(* Logix 5000 AddOnInstructionDefinition export SPEL_LocalGet; software revision 30.01 *)

ADD_ON_INSTRUCTION SPEL_ExecCmd   (* revision 1.2 *)
// Executes a command in the robot controller.  Normally this is called by higher level AOIs.
VAR_INPUT
   Start : BOOL; {required}
   MaxTime : DINT := 3000; {required}
END_VAR
VAR_OUTPUT
   InCycle : BOOL; {access Read Only, visible}
   Done : BOOL; {access Read Only, visible}
   Error : BOOL; {access Read Only, visible}
END_VAR
VAR_IN_OUT
   ExtInputs : AB:ETHERNET_MODULE_INT_128Bytes:I:0; {required}
        .DATA[0].0   // ExtCmdGet
        .DATA[0].1   // ExtRespSet
        .DATA[0].2   // ExtCmdResult
        .DATA[0].3   // ExtError
   ExtOutputs : AB:ETHERNET_MODULE_INT_128Bytes:O:0; {required}
        .DATA[0].0   // ExtCmdSet
        .DATA[0].1   // ExtRespGet
        .DATA[0].2   // ExtCmdReset
END_VAR
VAR_INPUT
   Cmd : INT; {required}
   CmdParam1 : INT; {required}
   CmdParam2 : INT; {required}
   CmdParam3 : INT; {required}
   CmdParam4 : INT; {required}
   CmdParam5 : INT; {required}
   CmdParam6 : INT; {required}
   CmdParam7 : INT; {required}
END_VAR
VAR_OUTPUT
   CmdEcho : INT; {access Read Only, visible}
   Resp1 : INT; {access Read Only, visible}
   Resp2 : INT; {access Read Only, visible}
   Resp3 : INT; {access Read Only, visible}
   Resp4 : INT; {access Read Only, visible}
   Resp5 : INT; {access Read Only, visible}
   Resp6 : INT; {access Read Only, visible}
   Resp7 : INT; {access Read Only, visible}
   ErrCode1 : INT; {access Read Only, visible}
   ErrCode2 : INT; {access Read Only, visible}
END_VAR
VAR
   ExtReset : BOOL; {access None}
   ExtError : BOOL; {access None}
   ExtCmdSet : BOOL; {access None}   // Cmd Ready
   ExtCmdGet : BOOL; {access None}   // Cmd Received
   CmdXferDone : BOOL; {access None}
   ExtRespSet : BOOL; {access None}   // Resp Ready
   RespXferDone : BOOL; {access None}
   ExtCmdResult : BOOL; {access None}   // Normal or Error?
   TmrCmdDataRdy : TIMER := (PRE := 5); {access None}
   OneShotDoneOff : BOOL; {access None}
   OneShotStart : BOOL; {access None}
   StartInit : BOOL; {access None}
   OneShotStartError : BOOL; {access None}
   TmrCycle : TIMER := (PRE := 5000); {access None}
   OneshotTmrPreset : BOOL; {access None}
   TmrCmdSet : TIMER := (PRE := 20); {access None}
   OnShotCmdDataXfer : BOOL; {access None}
   OneShotRespDataXfer : BOOL; {access None}
   OneShotDataRdy : BOOL; {access None}
   OtherCmdInCycle : BOOL; {access None}
   s : BOOL; {access None}
   OneShotUnsetCmdIncycle : BOOL; {access None}
   OneShotSetCmdIncycle : BOOL; {access None}
   OneShotSetOtherCmdInCycleError : BOOL; {access None}
   OneShotSetBit : BOOL; {access None}
   MaxTimeError : BOOL; {access None}
END_VAR

ROUTINE Logic   (* ladder *)
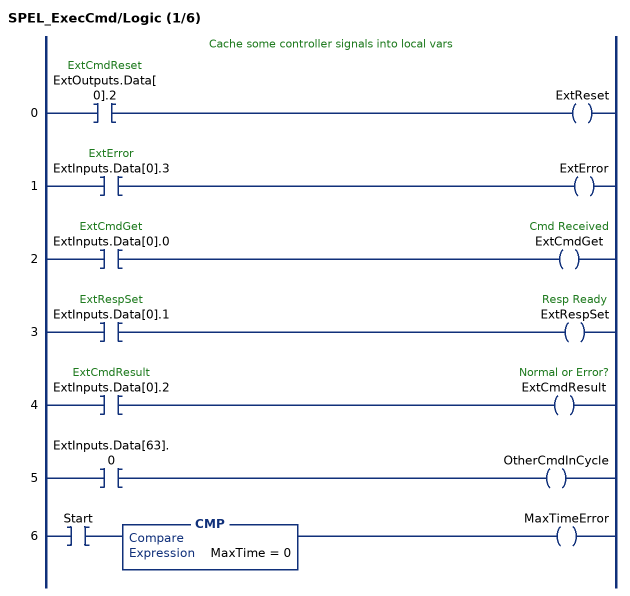
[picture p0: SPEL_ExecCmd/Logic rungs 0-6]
   // Cache some controller signals into local vars
   0: XIC(ExtOutputs.Data[0].2)OTE(ExtReset);
   1: XIC(ExtInputs.Data[0].3)OTE(ExtError);
   2: XIC(ExtInputs.Data[0].0)OTE(ExtCmdGet);
   3: XIC(ExtInputs.Data[0].1)OTE(ExtRespSet);
   4: XIC(ExtInputs.Data[0].2)OTE(ExtCmdResult);
   5: XIC(ExtInputs.Data[63].0)OTE(OtherCmdInCycle);
   6: XIC(Start)CMP(MaxTime = 0)OTE(MaxTimeError);
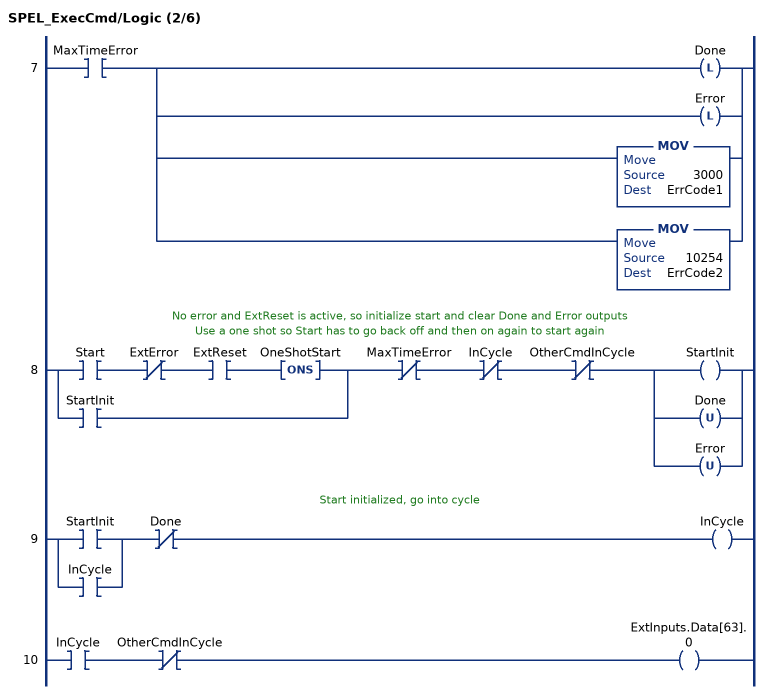
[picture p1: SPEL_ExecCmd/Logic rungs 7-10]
   7: XIC(MaxTimeError)[OTL(Done) ,OTL(Error) ,MOV(3000,ErrCode1) ,MOV(10254,ErrCode2) ];
   // No error and ExtReset is active, so initialize start and clear Done and Error outputs
   // Use a one shot so Start has to go back off and then on again to start again
   8: [XIC(Start) XIO(ExtError) XIC(ExtReset) ONS(OneShotStart) ,XIC(StartInit) ]XIO(MaxTimeError)XIO(InCycle)XIO(OtherCmdInCycle)[OTE(StartInit) ,OTU(Done) ,OTU(Error) ];
   // Start initialized, go into cycle
   9: [XIC(StartInit) ,XIC(InCycle) ]XIO(Done)OTE(InCycle);
   10: XIC(InCycle)XIO(OtherCmdInCycle)OTE(ExtInputs.Data[63].0);
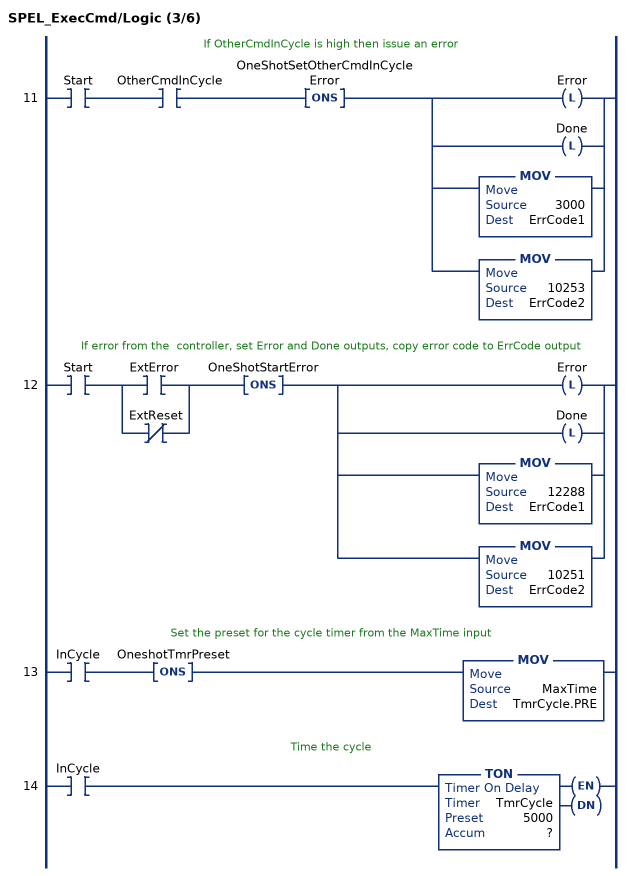
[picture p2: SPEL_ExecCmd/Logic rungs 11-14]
   // If OtherCmdInCycle is high then issue an error
   11: XIC(Start)XIC(OtherCmdInCycle)ONS(OneShotSetOtherCmdInCycleError)[OTL(Error) ,OTL(Done) ,MOV(3000,ErrCode1) ,MOV(10253,ErrCode2) ];
   // If error from the  controller, set Error and Done outputs, copy error code to ErrCode output
   12: XIC(Start)[XIC(ExtError) ,XIO(ExtReset) ]ONS(OneShotStartError)[OTL(Error) ,OTL(Done) ,MOV(12288,ErrCode1) ,MOV(10251,ErrCode2) ];
   // Set the preset for the cycle timer from the MaxTime input
   13: XIC(InCycle)ONS(OneshotTmrPreset)MOV(MaxTime,TmrCycle.PRE);
   // Time the cycle
   14: XIC(InCycle)TON(TmrCycle,?,?);
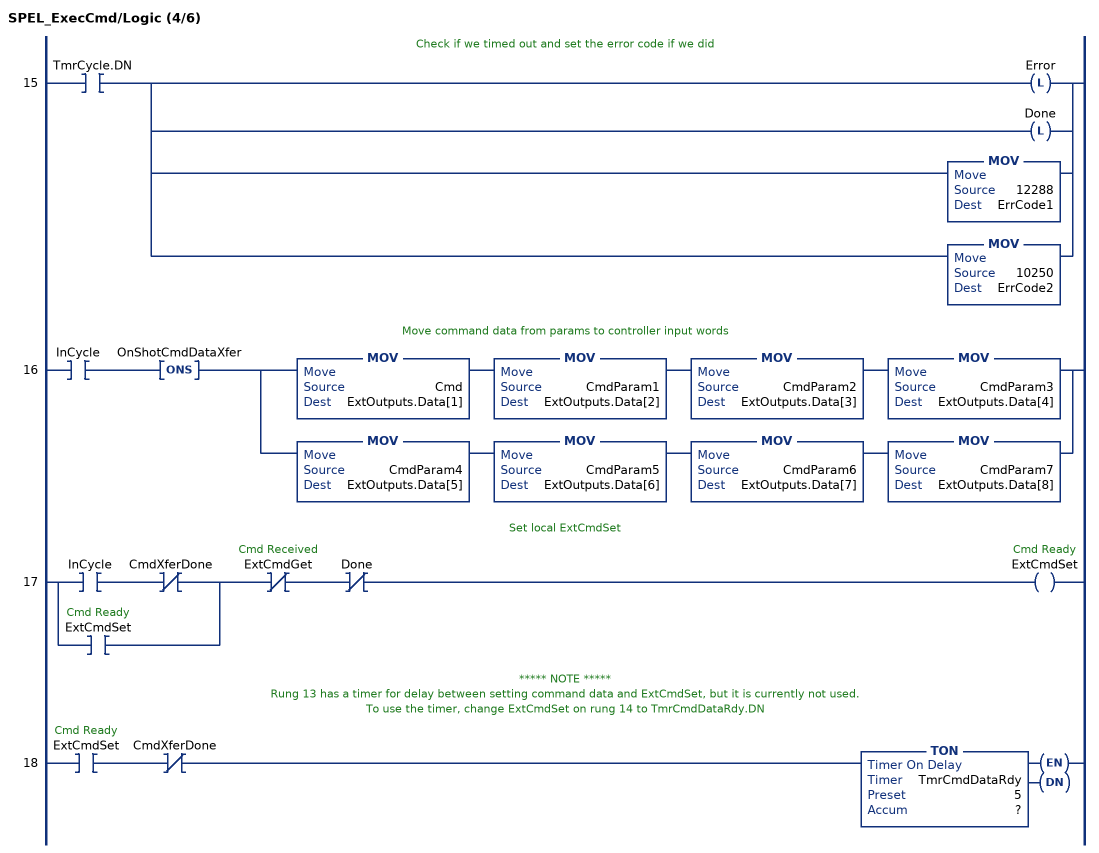
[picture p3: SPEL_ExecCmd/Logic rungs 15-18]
   // Check if we timed out and set the error code if we did
   15: XIC(TmrCycle.DN)[OTL(Error) ,OTL(Done) ,MOV(12288,ErrCode1) ,MOV(10250,ErrCode2) ];
   // Move command data from params to controller input words
   16: XIC(InCycle)ONS(OnShotCmdDataXfer)[MOV(Cmd,ExtOutputs.Data[1]) MOV(CmdParam1,ExtOutputs.Data[2]) MOV(CmdParam2,ExtOutputs.Data[3]) MOV(CmdParam3,ExtOutputs.Data[4]) ,MOV(CmdParam4,ExtOutputs.Data[5]) MOV(CmdParam5,ExtOutputs.Data[6]) MOV(CmdParam6,ExtOutputs.Data[7]) MOV(CmdParam7,ExtOutputs.Data[8]) ];
   // Set local ExtCmdSet
   17: [XIC(InCycle) XIO(CmdXferDone) ,XIC(ExtCmdSet) ]XIO(ExtCmdGet)XIO(Done)OTE(ExtCmdSet);
   // ***** NOTE *****
   // Rung 13 has a timer for delay between setting command data and ExtCmdSet, but it is currently not used.
   // To use the timer, change ExtCmdSet on rung 14 to TmrCmdDataRdy.DN
   18: XIC(ExtCmdSet)XIO(CmdXferDone)TON(TmrCmdDataRdy,?,?);
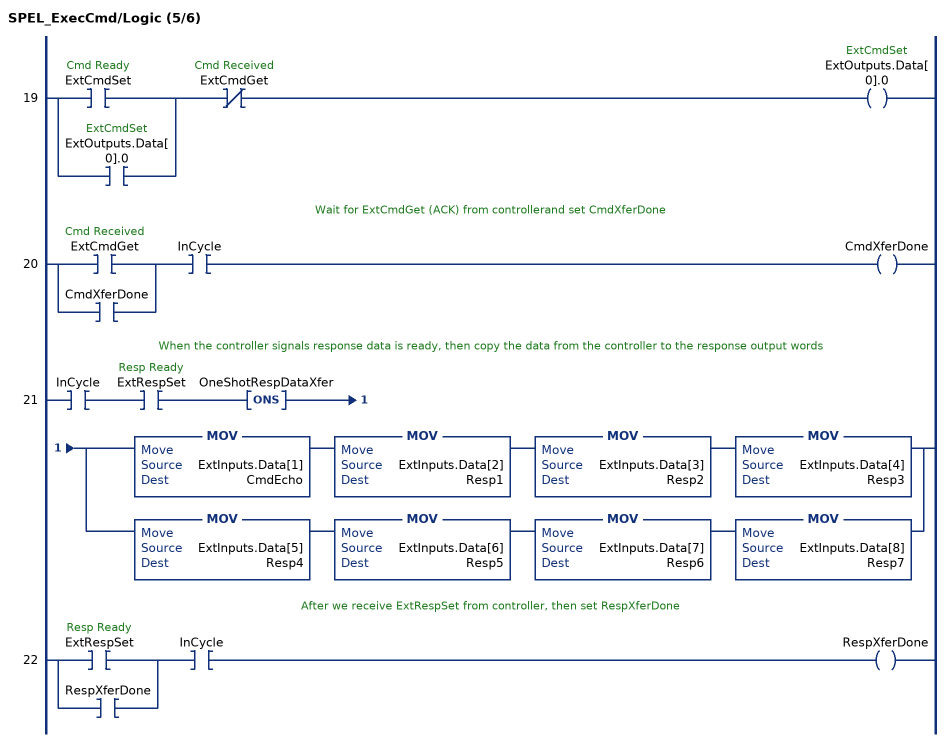
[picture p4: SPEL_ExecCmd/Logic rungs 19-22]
   19: [XIC(ExtCmdSet) ,XIC(ExtOutputs.Data[0].0) ]XIO(ExtCmdGet)OTE(ExtOutputs.Data[0].0);
   // Wait for ExtCmdGet (ACK) from controllerand set CmdXferDone
   20: [XIC(ExtCmdGet) ,XIC(CmdXferDone) ]XIC(InCycle)OTE(CmdXferDone);
   // When the controller signals response data is ready, then copy the data from the controller to the response output words
   21: XIC(InCycle)XIC(ExtRespSet)ONS(OneShotRespDataXfer)[MOV(ExtInputs.Data[1],CmdEcho) MOV(ExtInputs.Data[2],Resp1) MOV(ExtInputs.Data[3],Resp2) MOV(ExtInputs.Data[4],Resp3) ,MOV(ExtInputs.Data[5],Resp4) MOV(ExtInputs.Data[6],Resp5) MOV(ExtInputs.Data[7],Resp6) MOV(ExtInputs.Data[8],Resp7) ];
   // After we receive ExtRespSet from controller, then set RespXferDone
   22: [XIC(ExtRespSet) ,XIC(RespXferDone) ]XIC(InCycle)OTE(RespXferDone);
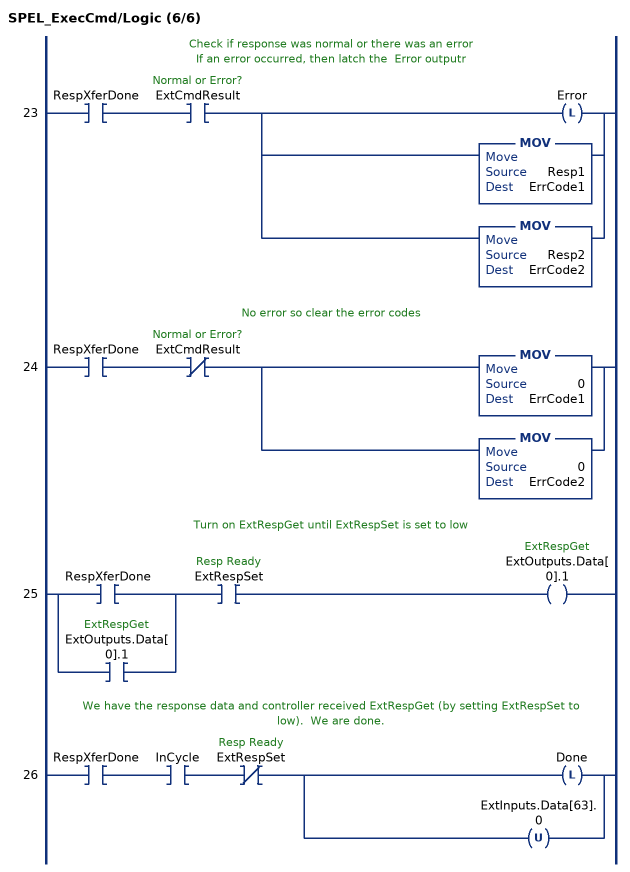
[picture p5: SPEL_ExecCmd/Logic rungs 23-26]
   // Check if response was normal or there was an error
   // If an error occurred, then latch the  Error outputr
   23: XIC(RespXferDone)XIC(ExtCmdResult)[OTL(Error) ,MOV(Resp1,ErrCode1) ,MOV(Resp2,ErrCode2) ];
   // No error so clear the error codes
   24: XIC(RespXferDone)XIO(ExtCmdResult)[MOV(0,ErrCode1) ,MOV(0,ErrCode2) ];
   // Turn on ExtRespGet until ExtRespSet is set to low
   25: [XIC(RespXferDone) ,XIC(ExtOutputs.Data[0].1) ]XIC(ExtRespSet)OTE(ExtOutputs.Data[0].1);
   // We have the response data and controller received ExtRespGet (by setting ExtRespSet to low).  We are done.
   26: XIC(RespXferDone)XIC(InCycle)XIO(ExtRespSet)[OTL(Done) ,OTU(ExtInputs.Data[63].0) ];
END_ROUTINE
END_ADD_ON_INSTRUCTION

ADD_ON_INSTRUCTION SPEL_LocalGet   (* revision 1.2, vendor SEIKO EPSON CORP. *)
// Gets the setting status of the Local coordinate system number.
VAR_INPUT
   Start : BOOL; {required}
END_VAR
VAR_OUTPUT
   InCycle : BOOL; {access Read Only, visible}
   Done : BOOL; {access Read Only, visible}
   Error : BOOL; {access Read Only, visible}
END_VAR
VAR_INPUT
   NumAxes : INT; {required}
   LocalNum : INT; {required}
END_VAR
VAR_OUTPUT
   LocalX : REAL; {visible}
   LocalY : REAL; {visible}
   LocalZ : REAL; {visible}
   LocalU : REAL; {visible}
   LocalV : REAL; {visible}
   LocalW : REAL; {visible}
END_VAR
VAR_IN_OUT
   ExtInputs : AB:ETHERNET_MODULE_INT_128Bytes:I:0; {required}
   ExtOutputs : AB:ETHERNET_MODULE_INT_128Bytes:O:0; {required}
END_VAR
VAR_OUTPUT
   ErrCode1 : INT; {access Read Only, visible}
   ErrCode2 : INT; {access Read Only, visible}
END_VAR
VAR
   Coordinatex1000 : DINT; {access None}
   Coordinate_INTS : INT[2]; {access None}
   ExecLocalGetZ : SPEL_ExecCmd := (MaxTime := 3000); {access None}
   ExecLocalGetY : SPEL_ExecCmd := (MaxTime := 3000); {access None}
   ExecLocalGetX : SPEL_ExecCmd := (MaxTime := 3000); {access None}
   X6 : BOOL; {access None}
   StartInit : BOOL[32]; {access None}
   OneShotStart : BOOL[32]; {access None}
   ExecLocalGetW : SPEL_ExecCmd := (MaxTime := 3000); {access None}
   ExecLocalGetV : SPEL_ExecCmd := (MaxTime := 3000); {access None}
   ExecLocalGetU : SPEL_ExecCmd := (MaxTime := 3000); {access None}
   ExecTimeout : DINT; {access None}
END_VAR

ROUTINE Logic   (* ladder *)
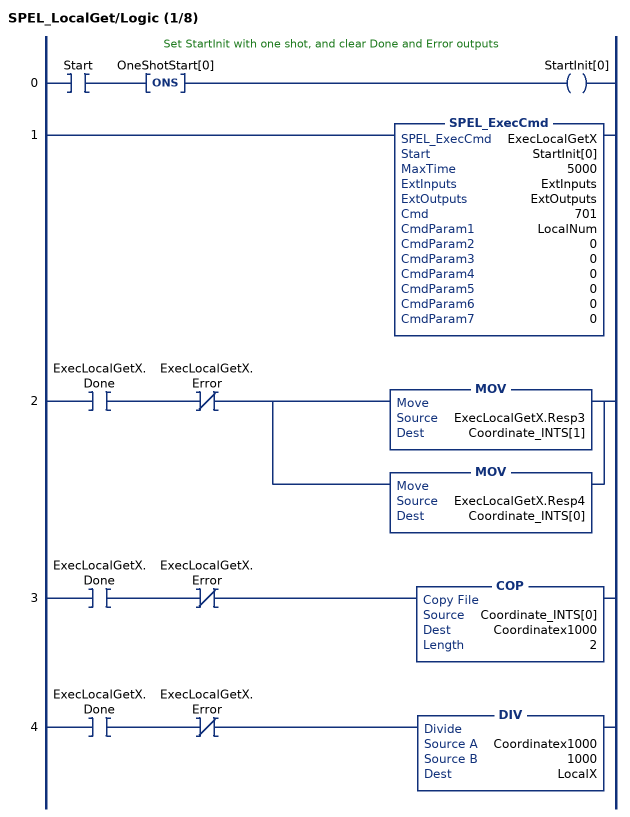
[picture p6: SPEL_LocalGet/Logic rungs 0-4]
   // Set StartInit with one shot, and clear Done and Error outputs
   0: XIC(Start)ONS(OneShotStart[0])OTE(StartInit[0]);
   1: SPEL_ExecCmd(ExecLocalGetX,StartInit[0],5000,ExtInputs,ExtOutputs,701,LocalNum,0,0,0,0,0,0);
   2: XIC(ExecLocalGetX.Done)XIO(ExecLocalGetX.Error)[MOV(ExecLocalGetX.Resp3,Coordinate_INTS[1]) ,MOV(ExecLocalGetX.Resp4,Coordinate_INTS[0]) ];
   3: XIC(ExecLocalGetX.Done)XIO(ExecLocalGetX.Error)COP(Coordinate_INTS[0],Coordinatex1000,2);
   4: XIC(ExecLocalGetX.Done)XIO(ExecLocalGetX.Error)DIV(Coordinatex1000,1000,LocalX);
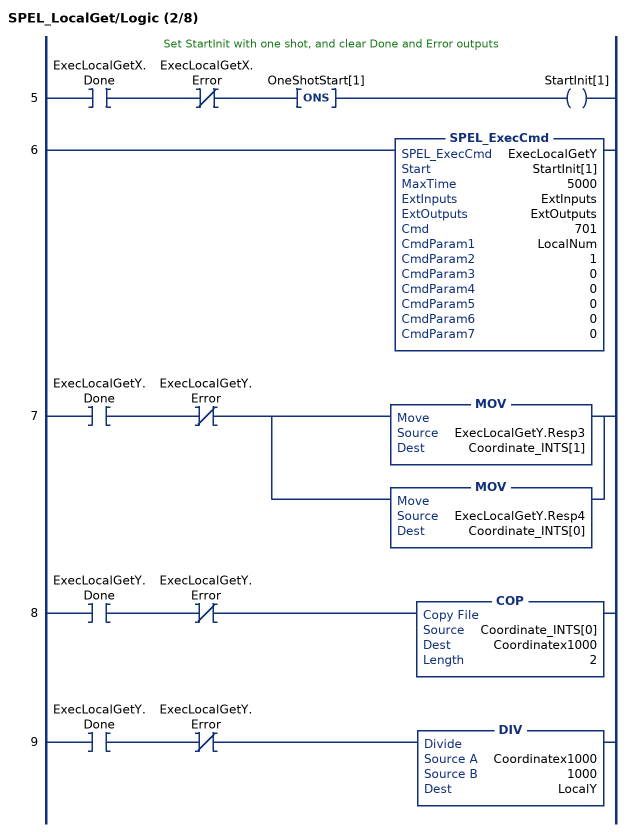
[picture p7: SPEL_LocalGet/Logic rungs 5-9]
   // Set StartInit with one shot, and clear Done and Error outputs
   5: XIC(ExecLocalGetX.Done)XIO(ExecLocalGetX.Error)ONS(OneShotStart[1])OTE(StartInit[1]);
   6: SPEL_ExecCmd(ExecLocalGetY,StartInit[1],5000,ExtInputs,ExtOutputs,701,LocalNum,1,0,0,0,0,0);
   7: XIC(ExecLocalGetY.Done)XIO(ExecLocalGetY.Error)[MOV(ExecLocalGetY.Resp3,Coordinate_INTS[1]) ,MOV(ExecLocalGetY.Resp4,Coordinate_INTS[0]) ];
   8: XIC(ExecLocalGetY.Done)XIO(ExecLocalGetY.Error)COP(Coordinate_INTS[0],Coordinatex1000,2);
   9: XIC(ExecLocalGetY.Done)XIO(ExecLocalGetY.Error)DIV(Coordinatex1000,1000,LocalY);
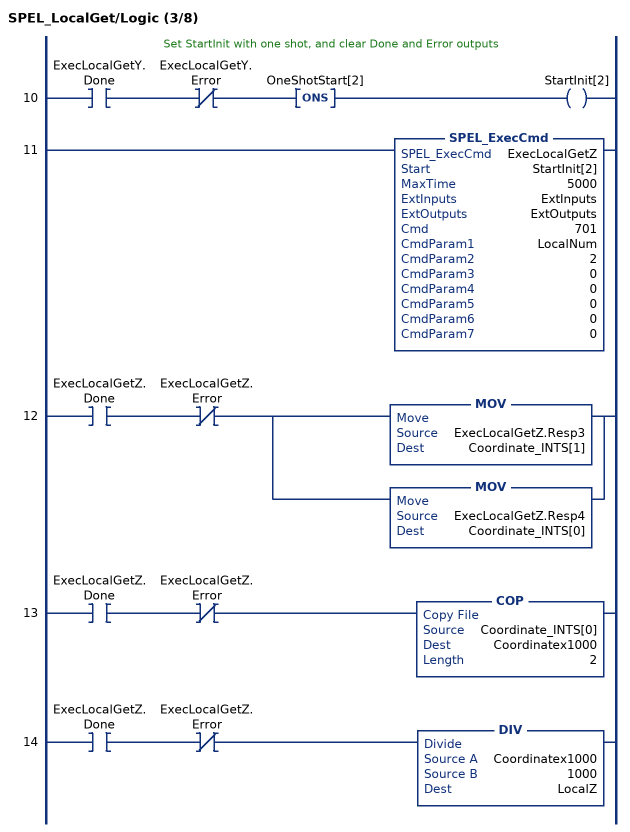
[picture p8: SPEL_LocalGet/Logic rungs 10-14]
   // Set StartInit with one shot, and clear Done and Error outputs
   10: XIC(ExecLocalGetY.Done)XIO(ExecLocalGetY.Error)ONS(OneShotStart[2])OTE(StartInit[2]);
   11: SPEL_ExecCmd(ExecLocalGetZ,StartInit[2],5000,ExtInputs,ExtOutputs,701,LocalNum,2,0,0,0,0,0);
   12: XIC(ExecLocalGetZ.Done)XIO(ExecLocalGetZ.Error)[MOV(ExecLocalGetZ.Resp3,Coordinate_INTS[1]) ,MOV(ExecLocalGetZ.Resp4,Coordinate_INTS[0]) ];
   13: XIC(ExecLocalGetZ.Done)XIO(ExecLocalGetZ.Error)COP(Coordinate_INTS[0],Coordinatex1000,2);
   14: XIC(ExecLocalGetZ.Done)XIO(ExecLocalGetZ.Error)DIV(Coordinatex1000,1000,LocalZ);
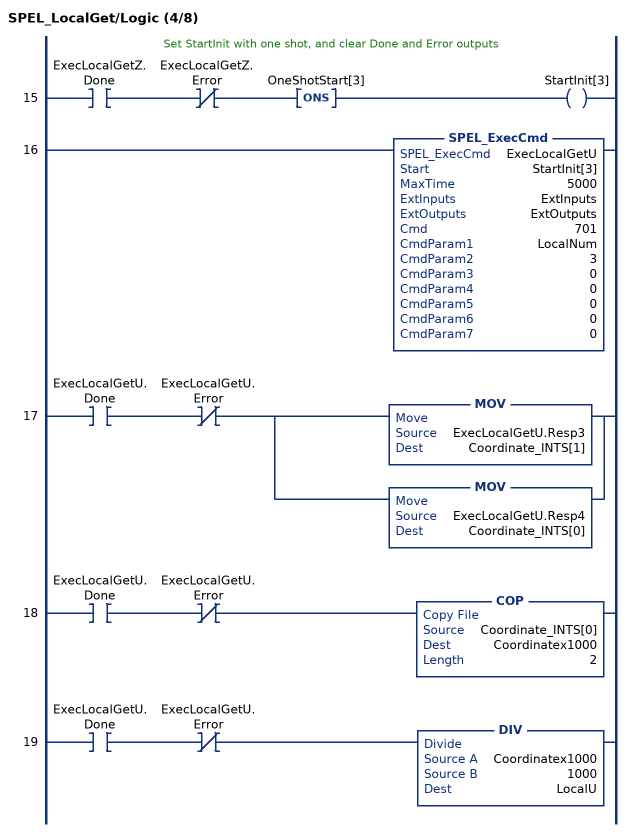
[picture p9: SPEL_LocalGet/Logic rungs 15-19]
   // Set StartInit with one shot, and clear Done and Error outputs
   15: XIC(ExecLocalGetZ.Done)XIO(ExecLocalGetZ.Error)ONS(OneShotStart[3])OTE(StartInit[3]);
   16: SPEL_ExecCmd(ExecLocalGetU,StartInit[3],5000,ExtInputs,ExtOutputs,701,LocalNum,3,0,0,0,0,0);
   17: XIC(ExecLocalGetU.Done)XIO(ExecLocalGetU.Error)[MOV(ExecLocalGetU.Resp3,Coordinate_INTS[1]) ,MOV(ExecLocalGetU.Resp4,Coordinate_INTS[0]) ];
   18: XIC(ExecLocalGetU.Done)XIO(ExecLocalGetU.Error)COP(Coordinate_INTS[0],Coordinatex1000,2);
   19: XIC(ExecLocalGetU.Done)XIO(ExecLocalGetU.Error)DIV(Coordinatex1000,1000,LocalU);
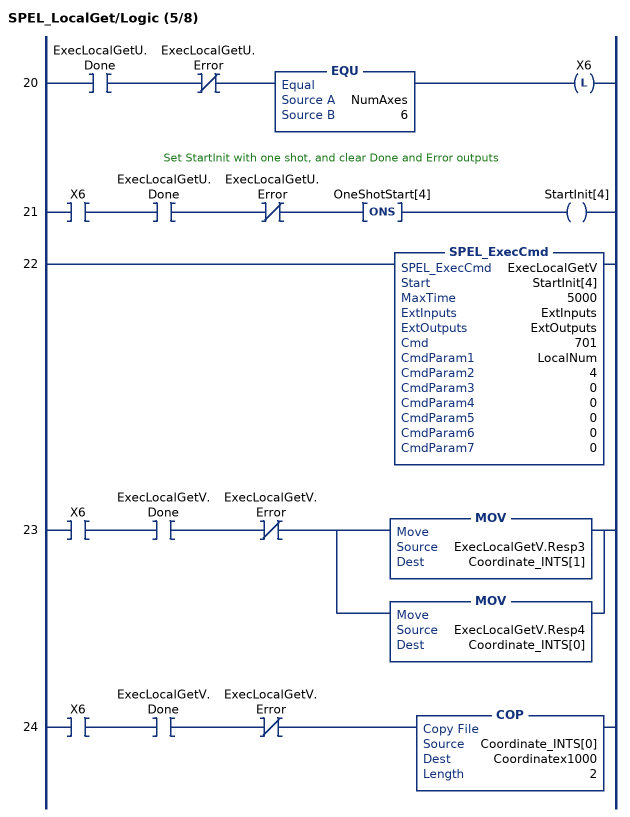
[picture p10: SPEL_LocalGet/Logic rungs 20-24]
   20: XIC(ExecLocalGetU.Done)XIO(ExecLocalGetU.Error)EQU(NumAxes,6)OTL(X6);
   // Set StartInit with one shot, and clear Done and Error outputs
   21: XIC(X6)XIC(ExecLocalGetU.Done)XIO(ExecLocalGetU.Error)ONS(OneShotStart[4])OTE(StartInit[4]);
   22: SPEL_ExecCmd(ExecLocalGetV,StartInit[4],5000,ExtInputs,ExtOutputs,701,LocalNum,4,0,0,0,0,0);
   23: XIC(X6)XIC(ExecLocalGetV.Done)XIO(ExecLocalGetV.Error)[MOV(ExecLocalGetV.Resp3,Coordinate_INTS[1]) ,MOV(ExecLocalGetV.Resp4,Coordinate_INTS[0]) ];
   24: XIC(X6)XIC(ExecLocalGetV.Done)XIO(ExecLocalGetV.Error)COP(Coordinate_INTS[0],Coordinatex1000,2);
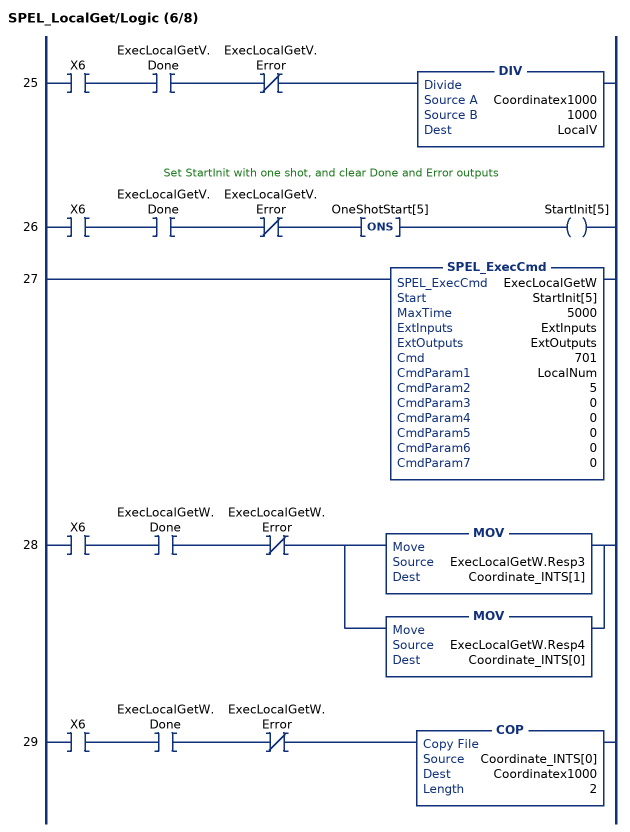
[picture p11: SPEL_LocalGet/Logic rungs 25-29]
   25: XIC(X6)XIC(ExecLocalGetV.Done)XIO(ExecLocalGetV.Error)DIV(Coordinatex1000,1000,LocalV);
   // Set StartInit with one shot, and clear Done and Error outputs
   26: XIC(X6)XIC(ExecLocalGetV.Done)XIO(ExecLocalGetV.Error)ONS(OneShotStart[5])OTE(StartInit[5]);
   27: SPEL_ExecCmd(ExecLocalGetW,StartInit[5],5000,ExtInputs,ExtOutputs,701,LocalNum,5,0,0,0,0,0);
   28: XIC(X6)XIC(ExecLocalGetW.Done)XIO(ExecLocalGetW.Error)[MOV(ExecLocalGetW.Resp3,Coordinate_INTS[1]) ,MOV(ExecLocalGetW.Resp4,Coordinate_INTS[0]) ];
   29: XIC(X6)XIC(ExecLocalGetW.Done)XIO(ExecLocalGetW.Error)COP(Coordinate_INTS[0],Coordinatex1000,2);
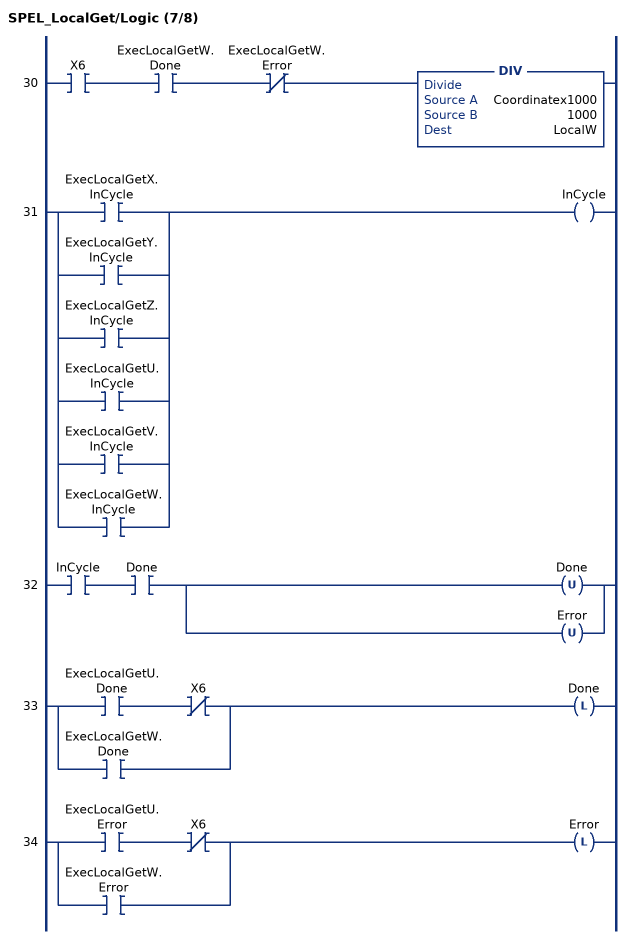
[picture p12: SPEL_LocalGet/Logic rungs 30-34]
   30: XIC(X6)XIC(ExecLocalGetW.Done)XIO(ExecLocalGetW.Error)DIV(Coordinatex1000,1000,LocalW);
   31: [XIC(ExecLocalGetX.InCycle) ,XIC(ExecLocalGetY.InCycle) ,XIC(ExecLocalGetZ.InCycle) ,XIC(ExecLocalGetU.InCycle) ,XIC(ExecLocalGetV.InCycle) ,XIC(ExecLocalGetW.InCycle) ]OTE(InCycle);
   32: XIC(InCycle)XIC(Done)[OTU(Done) ,OTU(Error) ];
   33: [XIC(ExecLocalGetU.Done) XIO(X6) ,XIC(ExecLocalGetW.Done) ]OTL(Done);
   34: [XIC(ExecLocalGetU.Error) XIO(X6) ,XIC(ExecLocalGetW.Error) ]OTL(Error);
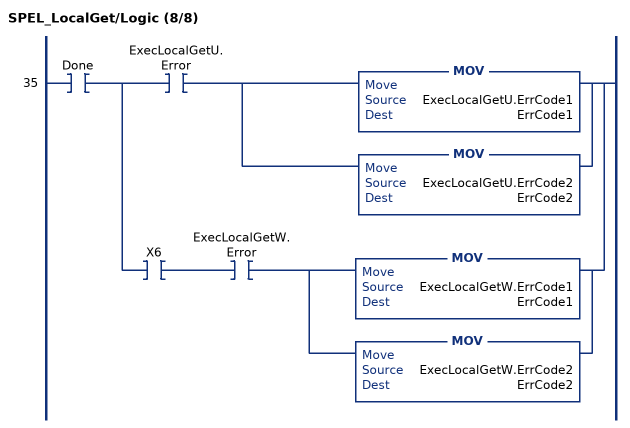
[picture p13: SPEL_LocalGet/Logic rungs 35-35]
   35: XIC(Done)[XIC(ExecLocalGetU.Error) [MOV(ExecLocalGetU.ErrCode1,ErrCode1) ,MOV(ExecLocalGetU.ErrCode2,ErrCode2) ] ,XIC(X6) XIC(ExecLocalGetW.Error) [MOV(ExecLocalGetW.ErrCode1,ErrCode1) ,MOV(ExecLocalGetW.ErrCode2,ErrCode2) ] ];
END_ROUTINE
END_ADD_ON_INSTRUCTION
